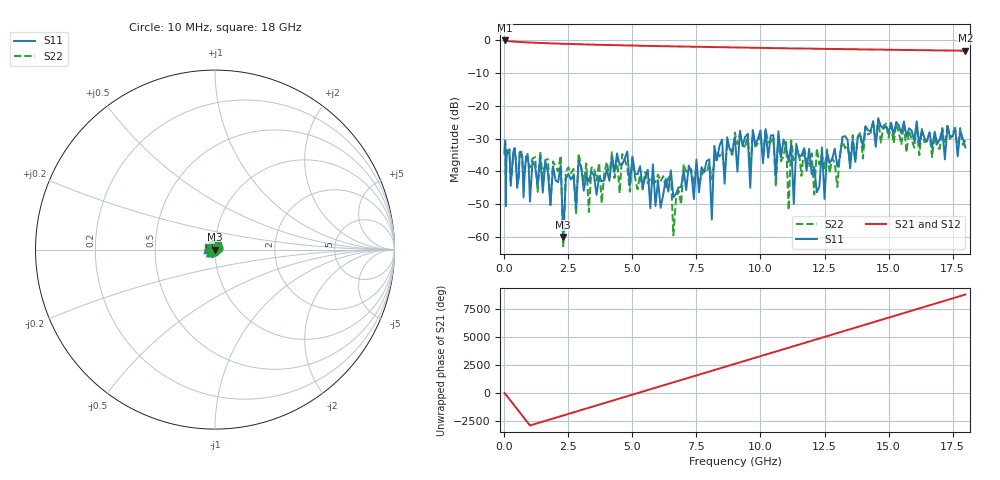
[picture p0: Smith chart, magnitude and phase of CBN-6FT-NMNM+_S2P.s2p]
!Mini-Circuits Laboratory
!S-Parameters
!Type: N-Type Cable
!Model: CBN-6FT-NMNM+
!S/N: Unit 001
!TEST CONDITIONS: Z:50 OHM SYSTEM, INPUT POWER = -10dBm, TEMP:25°C
!Run#: YH0987_QN252854 / Date Code: 2525
!Fixture: N/A, Pressing Arm: N/A
!Network Analyzer: Keysight P5028B;  Serial number: 82029
!Date: 8/1/2025 at 4:13:56 PM
!No.: Unit# 1 (001)
!Tested with:
# Hz  S  dB  R  50
!Frequency  S11 dB  S11 Deg  S21 dB  S21 Deg  S12 dB  S12 Deg  S22 dB  S22 Deg
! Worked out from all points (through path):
!   198 points, 10 MHz to 18 GHz, reference 50 ohm
!   highest |S21| = -0.07 dB at 10 MHz (marker M1); lowest = -3.2 dB at 18 GHz (marker M2)
!   lowest |S11| = -60.0 dB at 2.3 GHz (marker M3), VSWR 1.00, Z = 49.9 - j0.0405 ohm
!   |S11| at or under -10 dB: start of sweep to end of sweep
!   |S22| runs from -62.8 to -23.7 dB; largest |S21 - S12| = 0.00089
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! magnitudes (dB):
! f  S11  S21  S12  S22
! 10 MHz  -34.7  -0.1  -0.1  -34.6
! 60 MHz  -50.6  -0.2  -0.2  -49.2
! 90 MHz  -33.4  -0.2  -0.2  -33.5
! 1.8 GHz  -50.2  -1.0  -0.9  -50.2
! 2.2 GHz  -38.1  -1.1  -1.1  -35.2
! 2.3 GHz  -60.0  -1.1  -1.1  -62.8
! 2.4 GHz  -42.2  -1.1  -1.1  -40.1
! 3.1 GHz  -45.9  -1.3  -1.3  -43.2
! 4.8 GHz  -33.9  -1.6  -1.6  -38.9
! 6.1 GHz  -51.1  -1.8  -1.8  -43.0
! 6.5 GHz  -39.7  -1.9  -1.9  -40.6
! 6.6 GHz  -47.9  -1.9  -1.9  -59.5
! 7 GHz  -39.7  -1.9  -1.9  -37.7
! 8 GHz  -36.3  -2.1  -2.1  -37.6
! 8.1 GHz  -54.7  -2.1  -2.1  -42.3
! 8.2 GHz  -32.2  -2.1  -2.1  -37.3
! 9.1 GHz  -40.1  -2.2  -2.2  -31.7
! 12.1 GHz  -38.6  -2.6  -2.6  -47.0
! 12.2 GHz  -46.3  -2.6  -2.6  -33.0
! 13 GHz  -38.5  -2.7  -2.7  -44.7
! 15.1 GHz  -25.1  -2.9  -2.9  -26.1
! 18 GHz  -32.7  -3.2  -3.2  -30.5
